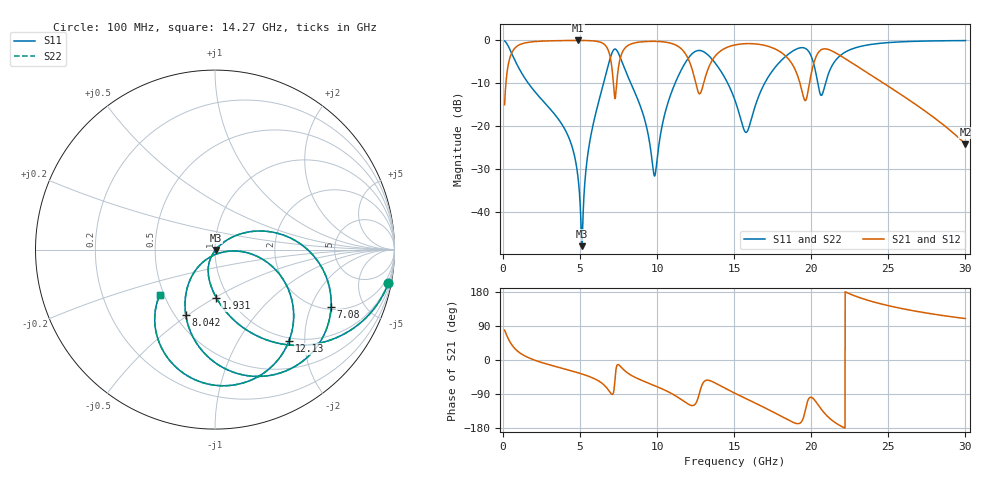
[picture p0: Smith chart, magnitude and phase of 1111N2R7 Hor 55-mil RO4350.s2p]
# GHz S MA R 50
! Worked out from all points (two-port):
!   3201 points, 100 MHz to 30 GHz, reference 50 ohm
!   highest |S21| = -0.04 dB at 4.837 GHz (marker M1); lowest = -24.2 dB at 30 GHz (marker M2)
!   |S21| within 3 dB of the highest: 550.5 MHz to 6.892 GHz (6.341 GHz wide, 170 % of centre); 13.93 GHz to 18.13 GHz (4.194 GHz wide, 26.2 % of centre)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
!   lowest |S11| = -48.0 dB at 5.118 GHz (marker M3), VSWR 1.01, Z = 50.3 - j0.232 ohm
!   |S11| at or under -10 dB: 1.635 GHz to 6.519 GHz (4.884 GHz wide, 120 % of centre); 8.287 GHz to 11.16 GHz (2.876 GHz wide, 29.6 % of centre); 14.58 GHz to 16.98 GHz (2.4 GHz wide, 15.2 % of centre)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
!   |S22| runs from -48.0 to -0.1 dB; largest |S21 - S12| = 0
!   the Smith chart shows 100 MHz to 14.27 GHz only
!   S11 on the Smith chart (normalised r, x): 100 MHz: 1, -10; 1.931 GHz: 0.88, -0.51; 7.08 GHz: 2.13, -2.82; 8.042 GHz: 0.57, -0.49; 12.13 GHz: 0.95, -1.68; 14.27 GHz: 0.47, -0.29
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0.1  0.984 -11.0  0.1777 79.0  0.1777 79.0  0.984 -11.0
1.931375  0.2692 -88.4  0.9618 1.4  0.9618 1.4  0.2692 -88.4
4.837281  0.02751 -116.8  0.9959 -33.4  0.9959 -33.4  0.02751 -116.8
5.089563  0.004808 -72.9  0.9955 -36.5  0.9955 -36.5  0.004808 -72.9
5.117594  0.003969 -35.5  0.9955 -36.9  0.9955 -36.9  0.003969 -35.5
5.687563  0.0758 39.2  0.989 -45.1  0.989 -45.1  0.0758 39.2
7.079781  0.7208 -26.2  0.4489 -90.8  0.4489 -90.8  0.7208 -26.2
8.042188  0.4 -114.0  0.8544 -33.1  0.8544 -33.1  0.4 -114.0
9.780125  0.02773 -88.1  0.9731 -66.8  0.9731 -66.8  0.02773 -88.1
10.06978  0.05273 -13.8  0.9699 -71.7  0.9699 -71.7  0.05273 -13.8
12.12541  0.6547 -51.0  0.5463 -118.7  0.5463 -118.7  0.6547 -51.0
12.77013  0.7607 -85.6  0.2381 -83.6  0.2381 -83.6  0.7607 -85.6
14.26512  0.3995 -140.5  0.7827 -71.6  0.7827 -71.6  0.3995 -140.5
15.05  0.1992 -147.6  0.8832 -87.9  0.8832 -87.9  0.1992 -147.6
15.81619  0.08515 -91.2  0.9149 -102.9  0.9149 -102.9  0.08515 -91.2
17.84378  0.5311 -63.8  0.7608 -144.1  0.7608 -144.1  0.5311 -63.8
19.58172  0.8098 -117.0  0.199 -138.1  0.199 -138.1  0.8098 -117.0
20.03956  0.6221 -140.4  0.4424 -99.1  0.4424 -99.1  0.6221 -140.4
20.63756  0.2279 -116.2  0.7746 -129.2  0.7746 -129.2  0.2279 -116.2
21.31031  0.4913 -82.2  0.7556 -157.9  0.7556 -157.9  0.4913 -82.2
25.01978  0.9411 -129.5  0.2895 143.2  0.2895 143.2  0.9411 -129.5
30  0.992 -163.7  0.06151 109.4  0.06151 109.4  0.992 -163.7
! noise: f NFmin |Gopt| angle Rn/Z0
0.1  0.001559  0.8908  3.144  0.003105
3.417  0.01033  0.5025  26.82  0.00342
6.743  0.1009  0.8786  47.62  0.1505
10.06  0.06905  0.7614  68.96  0.04023
13.39  0.3632  0.936  88.75  0.6481
16.7  0.1489  0.8217  106.3  0.06409
20.03  0.5702  0.9417  123.4  0.4937
23.35  0.2091  0.8328  137  0.0374
26.67  0.319  0.8844  150.9  0.04002
30  0.7261  0.9488  165.5  0.05279
